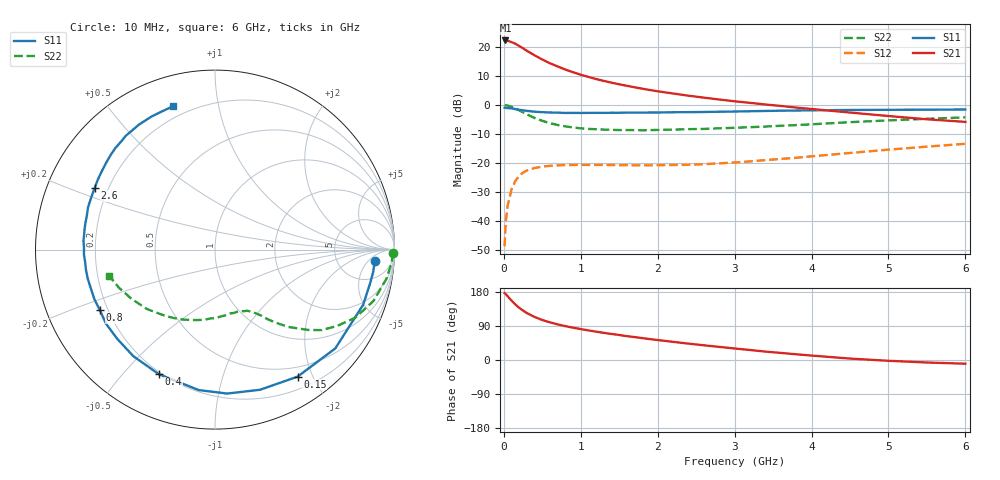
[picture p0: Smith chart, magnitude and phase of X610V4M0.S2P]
! SIEMENS Small Signal Semiconductors
! BFP193W
! Si NPN RF Bipolar Junction Transistor in SOT343
! VCE = 10 V  IC = 4 mA
! Common Emitter S-Parameters:  April 1994
# GHz  S  MA  R  50
!  f  S11  S21  S12  S22
! GHz  MAG  ANG  MAG  ANG  MAG  ANG  MAG  ANG
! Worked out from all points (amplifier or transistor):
!   40 points, 10 MHz to 6 GHz, reference 50 ohm
!   highest |S21| = 22.2 dB at 20 MHz (marker M1)
!   |S21| within 3 dB of that: start of sweep to 266.7 MHz
!   unconditionally stable (mu >= 1): 1.849 GHz to 4.637 GHz
!   at 200 MHz: K = 0.13, MSG = 22.3 dB, |S12| = -24.5 dB
!   at 1.5 GHz: K = 0.84, MSG = 13.9 dB, |S12| = -20.8 dB
!   at 6 GHz: K = 0.92, MSG = 3.8 dB, |S12| = -13.4 dB
!   S11 on the Smith chart (normalised r, x): 10 MHz: 13, -8; 150 MHz: 0.36, -1.79; 400 MHz: 0.19, -0.63; 800 MHz: 0.17, -0.24; 2.6 GHz: 0.15, +0.24; 6 GHz: 0.14, +0.74
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0.01  0.8926 -4.0  12.74 176.7  0.0037 86.3  0.993 -1.1
0.02  0.89 -8.1  12.81 175.1  0.0077 84.7  0.9867 -4.0
0.05  0.8808 -20.4  12.64 168.0  0.0186 78.9  0.9698 -9.5
0.1  0.8674 -39.4  12.01 156.8  0.0351 68.6  0.9279 -18.0
0.15  0.8441 -57.0  11.23 146.4  0.0491 60.1  0.8686 -25.9
0.2  0.8203 -72.2  10.27 137.6  0.0599 52.8  0.8037 -31.9
0.25  0.8049 -85.2  9.371 130.3  0.0682 46.8  0.7438 -37.1
0.3  0.7879 -96.6  8.497 123.8  0.0743 41.6  0.6851 -40.8
0.4  0.7616 -114.2  7.103 113.5  0.0819 34.1  0.5942 -46.5
0.5  0.7481 -127.5  6.024 105.5  0.0867 29.2  0.5305 -50.2
0.6  0.7375 -137.5  5.188 99.3  0.0892 25.5  0.4833 -53.1
0.7  0.7343 -145.8  4.573 94.0  0.0909 23.1  0.4499 -54.9
0.8  0.7248 -152.4  4.044 89.3  0.092 21.2  0.4258 -57.0
1.1  0.7273 -167.1  3.023 78.0  0.0926 18.1  0.3849 -62.2
1.3  0.7269 -174.6  2.577 71.6  0.0922 17.6  0.3753 -66.1
1.6  0.7346 176.0  2.124 62.9  0.0917 18.5  0.368 -71.8
2.2  0.7457 161.5  1.566 47.9  0.0922 23.6  0.3738 -84.8
2.6  0.7533 152.8  1.329 38.8  0.0953 28.3  0.3848 -94.0
3.2  0.7758 141.4  1.082 26.4  0.1064 34.6  0.4124 -107.8
4.5  0.8151 121.3  0.737 3.8  0.1485 40.8  0.5032 -138.8
5.5  0.8244 111.2  0.564 -6.6  0.1909 38.9  0.5753 -158.3
6  0.8319 106.3  0.509 -9.8  0.2137 37.1  0.6085 -166.2
